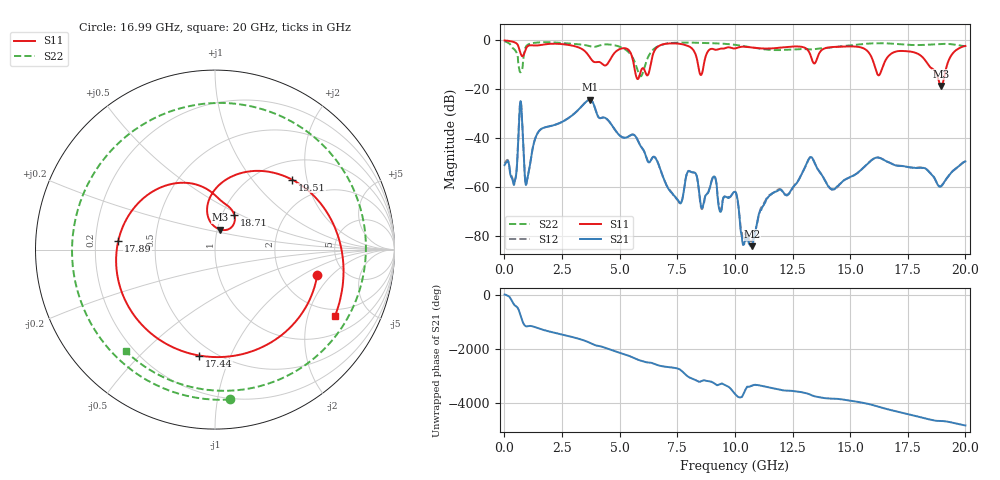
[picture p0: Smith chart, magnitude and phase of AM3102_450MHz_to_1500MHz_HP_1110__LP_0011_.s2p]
!Agilent Technologies,E8364B,MY43040894,A.07.50.67
!Agilent E8364B: A.07.50.67
!Date: Thursday, January 11, 2018 06:42:53
!Correction: S11(Full 2 Port(1,2))
!S21(Full 2 Port(1,2))
!S12(Full 2 Port(1,2))
!S22(Full 2 Port(1,2))
!S2P File: Measurements: S11, S21, S12, S22:
# Hz S  dB  R 50
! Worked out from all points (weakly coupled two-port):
!   1601 points, 10 MHz to 20 GHz, reference 50 ohm
!   highest |S21| = -24.35 dB at 3.708 GHz (marker M1); lowest = -84.2 dB at 10.74 GHz (marker M2)
!   lowest |S11| = -18.7 dB at 18.95 GHz (marker M3), VSWR 1.26, Z = 51.6 + j11.7 ohm
!   |S11| at or under -10 dB: 5.617 GHz to 6.345 GHz (727.7 MHz wide, 12.2 % of centre); 16.05 GHz to 16.45 GHz (401.3 MHz wide, 2.47 % of centre); 18.38 GHz to 19.21 GHz (823.8 MHz wide, 4.38 % of centre)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
!   |S22| runs from -14.8 to -0.4 dB; largest |S21 - S12| = 0.0014
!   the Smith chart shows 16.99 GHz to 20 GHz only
!   S11 on the Smith chart (normalised r, x): 16.99 GHz: 3.21, -1.37; 17.44 GHz: 0.42, -0.77; 17.89 GHz: 0.30, +0.04; 18.71 GHz: 1.14, +0.47; 19.51 GHz: 1.39, +1.63; 20 GHz: 1.68, -3.00
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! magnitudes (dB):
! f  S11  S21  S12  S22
! 10 MHz  -0.1  -51.0  -50.3  -0.4
! 447.3 MHz  -0.9  -57.8  -57.6  -3.9
! 697.2 MHz  -5.2  -24.9  -24.9  -13.1
! 972 MHz  -2.9  -57.9  -57.6  -2.1
! 1.497 GHz  -2.1  -37.2  -37.2  -0.9
! 3.346 GHz  -3.5  -27.1  -27.1  -1.8
! 3.708 GHz  -7.0  -24.3  -24.4  -2.4
! 6.682 GHz  -2.5  -50.6  -50.6  -2.4
! 7.594 GHz  -1.4  -66.2  -66.6  -1.0
! 8.031 GHz  -2.6  -53.6  -53.5  -1.0
! 10.01 GHz  -3.4  -62.0  -61.9  -1.9
! 10.74 GHz  -3.0  -84.2  -81.9  -3.0
! 13.34 GHz  -7.8  -47.9  -48.0  -3.8
! 14.24 GHz  -2.8  -61.0  -61.0  -2.9
! 16.68 GHz  -6.4  -49.9  -49.9  -1.3
! 16.99 GHz  -4.6  -51.2  -51.1  -1.5
! 17.44 GHz  -4.5  -51.7  -51.7  -1.8
! 17.89 GHz  -5.3  -52.2  -52.1  -2.0
! 18.71 GHz  -13.0  -57.4  -57.3  -1.6
! 18.95 GHz  -18.7  -59.8  -59.5  -1.5
! 19.51 GHz  -4.7  -53.0  -53.1  -1.8
! 20 GHz  -2.3  -49.5  -49.5  -2.5
